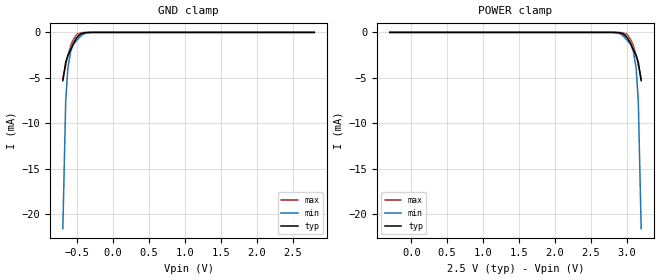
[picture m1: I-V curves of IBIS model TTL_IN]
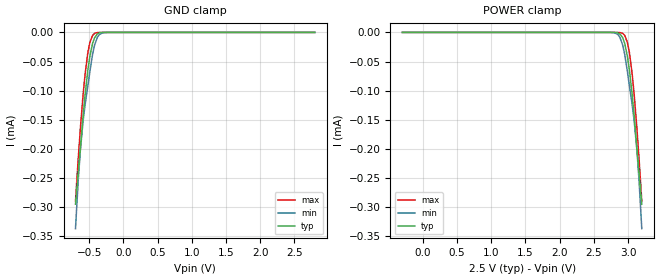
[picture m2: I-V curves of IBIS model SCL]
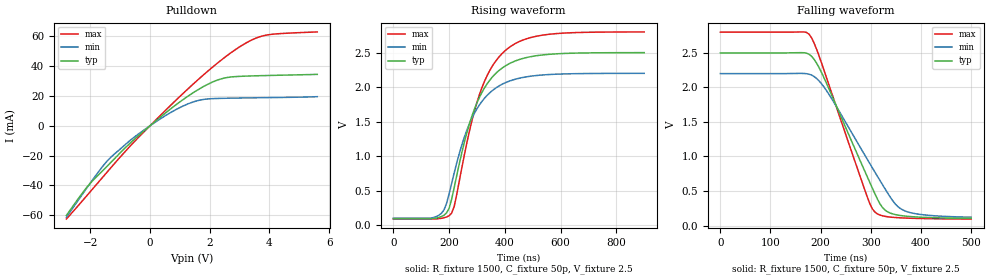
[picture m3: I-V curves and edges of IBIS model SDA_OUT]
[IBIS Ver]   3.2
[Comment Char]   |_char
[File name]   pca9530_2_5v.ibs
[File Rev]   1
[Date]   Nov 19, 2008 3:45:29 PM
[Source]
Generated by Seshadri Venkataramanan using IBIS Toolkit at NXP Tempe
[Notes]
[Disclaimer]
(C) Copyright 2007 NXP Semiconductors
All rights reserved
NXP Semiconductors (NXP) does not warrant that this model and any other
accompanying information (Model) accurately or fully represents the
operating characteristics and specifications of the semiconductor
products to which the Model relates.  Moreover, the Model is furnished
on an "as is" and with "all faults" basis, and without support or
warranty of any kind.  NXP disclaims all warranties, whether expressed
or implied or statutory, including without limitation all implied
warranties of non-infringement, merchantability and fitness for any
purpose, and those arising from a course of dealing or usage of trade.
NXP does not convey any license under its or any third party's patents,
copyrights or other intellectual property or proprietary rights.
You and your company assume any and all risks and liability arising out
of the application or use of the Model.
In no event shall NXP be liable for any direct, indirect, special,
consequential or incidental damages, however caused, whether in
warranty, contract or tort (including negligence), strict liability or
other legal theory, including, without limitation, for lost profits,
business interruption, or corruption or loss of data or information,
arising out of or in connection with the use of or the inability to use
the Model, even if NXP has been advised of the possibility of such
damages.
NXP provides the Model as a courtesy to our customers. You and your
company shall not distribute, convey, sell, or give the Model to anyone
else without receiving prior written permission from NXP.
NXP reserves the right to make changes without notice to the Model to
improve reliability, function, or design.
Please be aware that your receipt and subsequent use of the Model shall
serve as acceptance of these terms and conditions.  If you do not
accept these terms, return or destroy the Model immediately.
[Copyright]
2008
[Component]   PCA9530D
Si_location Pin
Timing_location Pin
[Manufacturer]   NXP Semiconductors
[Package]
R_pkg   4.81E-02   4.14E-02   5.47E-02
L_pkg   1.88E-09   1.54E-09   2.21E-09
C_pkg   4.49E-13   4.17E-13   4.81E-13
[Pin] signal_name   model_name   R_pin   L_pin   C_pin
1   A0   TTL_IN   5.47E-02  2.21E-09  4.81E-13
2   LED0   LED_OUT   4.14E-02  1.54E-09  4.20E-13
3   LED1   LED_OUT   4.14E-02  1.55E-09  4.20E-13
4   Vss   GND   5.47E-02  2.21E-09  4.80E-13
5   RESETb   TTL_IN   5.47E-02  2.21E-09  4.78E-13
6   SCL   SCL   4.14E-02  1.55E-09  4.17E-13
7   SDA   SDA   4.14E-02  1.54E-09  4.17E-13
8   VDD   POWER   5.47E-02  2.21E-09  4.79E-13
[Component]   PCA9530DP
Si_location Pin
Timing_location Pin
[Manufacturer]   NXP Semiconductors
[Package]
R_pkg   33.7m   30.1m   37.3m
L_pkg   1.74n   1.67n   1.81n
C_pkg   0.428p   0.422p   0.434p
[Pin] signal_name   model_name   R_pin   L_pin   C_pin
1   A0   TTL_IN   37.3m   1.81nH   0.428pF
2   LED0   LED_OUT   30.1m   1.67nH   0.422pF
3   LED1   LED_OUT   30.1m   1.67nH   0.428pF
4   Vss   GND   37.3m   1.81nH   0.434pF
5   RESETb   TTL_IN   37.3m   1.81nH   0.428pF
6   SCL   SCL   30.1m   1.67nH   0.422pF
7   SDA   SDA   30.1m   1.67nH   0.428pF
8   VDD   POWER   37.3m   1.81nH   0.434pF
[Model Selector]   SDA
SDA_IN   SDA Input
SDA_OUT   SDA output
| Models and submodels in the file (5): TTL_IN (Input), SCL (Input), SDA_OUT (Open_drain), LED_OUT (Open_drain), SDA_IN (Input)
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[Model]   TTL_IN
Model_type Input
Vinh=1.75
Vinl=0.75
C_comp   1.73p   1.7p   1.75p
[Temperature Range] 27   85   -40
[Voltage Range]   2.5   2.2   2.8
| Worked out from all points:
|   GND clamp passes 1 mA (typ) near -0.54 V on its own axis
[GND Clamp]
-700mV    -5.302mA   -21.58mA   -5.122mA
-660mV    -3.272mA   -7.517mA   -3.572mA
-630mV    -2.557mA   -3.927mA   -2.533mA
-590mV    -1.874mA   -2.048mA   -1.45mA
-560mV    -1.338mA   -1.435mA   -871.3uA
-520mV    -741.9uA   -984.4uA   -378uA
-490mV    -435.8uA   -731.4uA   -173.7uA
-450mV    -185.2uA   -388.2uA   -49.68uA
-380mV    -26uA      -81.86uA   -3.405uA
-280mV    -688.2nA   -3.733uA   -36.48nA
2.8V      51pA       210.6pA    36.58pA
[POWER Clamp]
-300mV    51pA       210.6pA    36.58pA
2.78V     -688.2nA   -3.733uA   -36.48nA
2.88V     -26uA      -81.86uA   -3.405uA
2.95V     -185.2uA   -388.2uA   -49.68uA
2.99V     -435.8uA   -731.4uA   -173.7uA
3.02V     -741.9uA   -984.4uA   -378uA
3.06V     -1.338mA   -1.435mA   -871.3uA
3.09V     -1.874mA   -2.048mA   -1.45mA
3.13V     -2.557mA   -3.927mA   -2.533mA
3.16V     -3.272mA   -7.517mA   -3.572mA
3.2V      -5.302mA   -21.58mA   -5.122mA
[Model]   SCL
Model_type Input
Vinh=1.75
Vinl=0.75
C_comp   3p   2.8p   3.2p
[Temperature Range] 27   85   -40
[Voltage Range]   2.5   2.2   2.8
[GND Clamp]
-700mV    -295uA     -337uA     -289.5uA
-660mV    -241.9uA   -254.1uA   -216.6uA
-630mV    -200.9uA   -204uA     -166.8uA
-590mV    -145.3uA   -153.2uA   -108.4uA
-560mV    -107.6uA   -124.5uA   -71.97uA
-520mV    -65.58uA   -92.63uA   -35.3uA
-490mV    -41.22uA   -67.38uA   -17.26uA
-450mV    -18.67uA   -37.44uA   -5.001uA
-420mV    -8.79uA    -21.47uA   -1.619uA
-350mV    -920.5nA   -3.647uA   -77.68nA
-210mV    -3.652nA   -27.14nA   -101.2pA
2.8V      6.71pA     20.63pA    5.609pA
[POWER Clamp]
-300mV    6.71pA     20.63pA    5.609pA
2.71V     -3.652nA   -27.14nA   -101.2pA
2.85V     -920.5nA   -3.647uA   -77.68nA
2.92V     -8.79uA    -21.47uA   -1.619uA
2.95V     -18.67uA   -37.44uA   -5.001uA
2.99V     -41.22uA   -67.38uA   -17.26uA
3.02V     -65.58uA   -92.63uA   -35.3uA
3.06V     -107.6uA   -124.5uA   -71.97uA
3.09V     -145.3uA   -153.2uA   -108.4uA
3.13V     -200.9uA   -204uA     -166.8uA
3.16V     -241.9uA   -254.1uA   -216.6uA
3.2V      -295uA     -337uA     -289.5uA
[Model]   SDA_OUT
Model_type Open_drain
Vref=2.5
Vmeas=1.25
Rref=1.5k
Cref=50p
C_comp   4p   3.8p   4.2p
[Temperature Range] 27   85   -40
[Voltage Range]   2.5   2.2   2.8
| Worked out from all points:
|   slope of the pulldown table from 0 to 0.375 V, typ, clamps not added: 59.7 ohm
|   falling waveform, R_fixture 1500, C_fixture 50p, V_fixture 2.5: 20-80 % time 86.5ns typ, 102ns min, 76.1ns max; typ from 2.5 V to 0.103 V
|   rising waveform, R_fixture 1500, C_fixture 50p, V_fixture 2.5: 20-80 % time 112ns typ, 111ns min, 112ns max; typ from 0.094 V to 2.5 V
[Pulldown]
-2.8V     -60.13mA   -61.4mA    -62.52mA
-2.04V    -39.46mA   -39.58mA   -45.13mA
-1.36V    -25.58mA   -22.05mA   -29.28mA
-340mV    -5.824mA   -4.817mA   -6.862mA
420mV     7.012mA    5.598mA    8.404mA
1.02V     16.3mA     12.42mA    20.04mA
1.61V     24.23mA    16.95mA    30.94mA
2.29V     30.87mA    18.35mA    42.54mA
2.72V     32.75mA    18.53mA    49.11mA
3.39V     33.43mA    18.75mA    57.39mA
3.99V     33.75mA    18.91mA    61.13mA
5.6V      34.48mA    19.53mA    62.94mA
[Falling Waveform]
R_fixture=1500
C_fixture=50p
V_fixture=2.5
V_fixture_min=2.2
V_fixture_max=2.8
0s        2.5V       2.2V       2.8V
176.8ns   2.481V     2.192V     2.771V
191.9ns   2.351V     2.129V     2.552V
212.1ns   2.052V     1.948V     2.131V
292.9ns   705.4mV    958.7mV    412.9mV
308.1ns   460mV      773.8mV    195.3mV
328.3ns   223.3mV    531.7mV    132.8mV
348.5ns   158.8mV    313.8mV    115.9mV
363.6ns   140.5mV    225.5mV    109.4mV
500ns     103.4mV    119.8mV    93.84mV
[Rising Waveform]
R_fixture=1500
C_fixture=50p
V_fixture=2.5
V_fixture_min=2.2
V_fixture_max=2.8
0s        94.33mV    101.4mV    89.58mV
163.6ns   112.5mV    144.7mV    95.01mV
181.8ns   144.8mV    221.7mV    107.5mV
209.1ns   375.5mV    604.5mV    173.9mV
263.6ns   1.337V     1.376V     1.191V
309.1ns   1.854V     1.744V     1.895V
354.5ns   2.143V     1.948V     2.301V
418.2ns   2.345V     2.09V      2.583V
563.6ns   2.477V     2.183V     2.768V
900ns     2.5V       2.2V       2.8V
[Ramp]
R_load=1500
dV/dt_r   1.443E+0/6.014E-8   1.431E+0/5.960E-8   1.452E+0/6.015E-8
dV/dt_f   1.442E+0/8.563E-8   1.428E+0/1.139E-7   1.452E+0/6.771E-8
|[End   SDA_OUT
